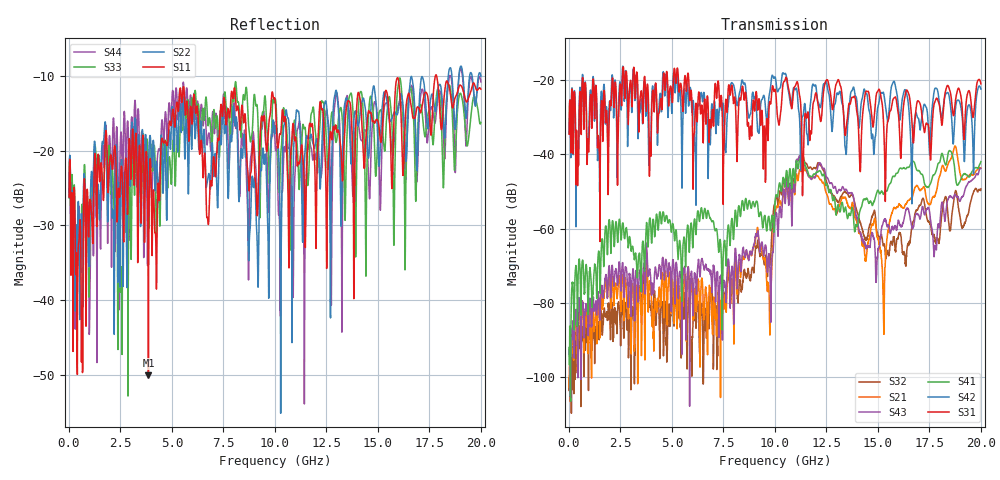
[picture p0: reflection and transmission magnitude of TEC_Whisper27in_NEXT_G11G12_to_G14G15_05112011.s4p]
! Tyco Electronics
! G11G12-G14G15_NEXT
!! PART DESCRIPTION: Whisper 27in Megtron 6 VLP-HVLP-VLP Channel Model, bulkhead 2.4mm test pts
!! MODEL DESCRIPTION: System 4-port S-parameter
!! MODEL STATUS: Measured
!! MODEL GEOMETRY: Channel Model
!! MODEL FREQUENCY RANGE: DC to 20.000 GHz in 10.000 MHz frequency steps
!! MODEL EDGE RATE LIMITATION: 25.00 ps (Using conservative 0.5/Fmax rule of thumb)
!! TIME-DOMAIN TRANSFORM CAUTIONS:
!! 1.) Do not simulate transient edge rates faster than the number listed above.  Edge rates faster than this number
!!  contain significant spectral content at frequencies above the model's highest frequency.
!! 2.) Even when simulating edge rates that are slower than the number listed above, be aware that the best time
!!  resolution possible with a direct iFFT is (1 / 2Fmax).  As a result, time resolution is typically not adequate
!!  for most time-domain simulations unless tricks such as windowing are used to minimize leakage and aliasing.
!! 3.) Because the model has a uniform frequency step, a direct iFFT will result in an impulse that that has a time
!!  length given by either (1 / Fstep) or (1 / 2Fstep), depending on the transform being used.  Care has been taken
!!  in selecting the frequency step to ensure a settled impulse response for the model.  Therefore, convolution with
!!  the model's impulse response should present no issues.  However, if directly concatenating s-parameter models
!!  in the frequency domain a user must either interpolate necessary interim frequencies or complete impulse response
!!  zero-padding.  Impulse response zero-padding is more difficult, but more accurate.
!! PORT DEFINITIONS:
!! Port  1  ----->  Side A  G11  G14  Side A  <-----  Port  2
!! Port  3  ----->  Side A  G12  G15  Side A  <-----  Port  4
! Point-to-Point link (differential)  !
! Connectors:  !
!  1: STRADA Whisper  !
! Materials:  !
!  Backplane: Megtron-6 HVLP  !
!  Daughtercard: Megtron-6 VLP  !
! Stack-up:  !
!  Backplane: 20 layers, 200mil thick  !
!  Daughtercard: 14 layers, 110mil thick  !
! Trace Length:  !
!  Backplane: 17in  !
!  Daightercards: 5in  !
! Trace Width:  !
!  Backplane: 8-13-8 mils  !
!  Daughtercards: 6-9-6 mils  !
! Geometry:  !
!  Backplane: Stripline  !
!  Daughtercards: Stripline  !
! Freq. Range: 0 GHz - 20 GHz  !
! Note1: non-mixed-mode s-parameters  !
! Note2: channel includes 2.4mm test points  !
! Created Wed May 11 15:00:19 2011
! 4 Port Network Data from SP1.SP block
! freq  magS11  angS11  magS12  angS12  magS13  angS13  magS14  angS14
!  magS21  angS21  magS22  angS22  magS23  angS23  magS24  angS24
!  magS31  angS31  magS32  angS32  magS33  angS33  magS34  angS34
!  magS41  angS41  magS42  angS42  magS43  angS43  magS44  angS44
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# hz S ma R 50
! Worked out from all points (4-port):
!   2000 points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, 10 MHz to 20 GHz, reference 50 ohm
!   strongest paths, dB at 10 MHz, 5.01 GHz, 10.01 GHz, 15.01 GHz, 20 GHz:
!     S31: -34.6, -25.4, -22.5, -22.8, -21.0
!     S42: -34.4, -27.8, -19.1, -27.0, -22.4
!     S41: -92.0, -59.5, -52.8, -49.7, -42.0
!     S43: -93.9, -71.1, -57.2, -65.8, -43.8
!     S21: -102.6, -73.8, -55.7, -63.1, -43.7
!     S32: -100.1, -78.6, -52.9, -61.7, -49.3
!   lowest |S11| = -50.0 dB at 3.86 GHz (marker M1), VSWR 1.01, Z = 49.7 - j0.123 ohm
!   |S11| at or under -10 dB: start of sweep to 17.8 GHz; 17.85 GHz to end of sweep
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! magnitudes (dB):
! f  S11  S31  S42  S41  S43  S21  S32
! 10 MHz  -26.2  -34.6  -34.4  -92.0  -93.9  -102.6  -100.1
! 3.86 GHz  -50.0  -25.3  -35.7  -63.0  -71.8  -81.1  -77.5
! 9.72 GHz  -16.0  -27.1  -24.2  -57.2  -67.1  -77.5  -67.4
! 11.27 GHz  -19.6  -28.4  -38.0  -42.0  -40.6  -44.7  -41.0
! 15.27 GHz  -14.4  -30.9  -23.4  -50.8  -58.1  -81.8  -64.6
! 15.8 GHz  -14.5  -24.8  -20.4  -46.0  -59.6  -54.3  -62.9
! 20 GHz  -11.8  -21.0  -22.4  -42.0  -43.8  -43.7  -49.3
